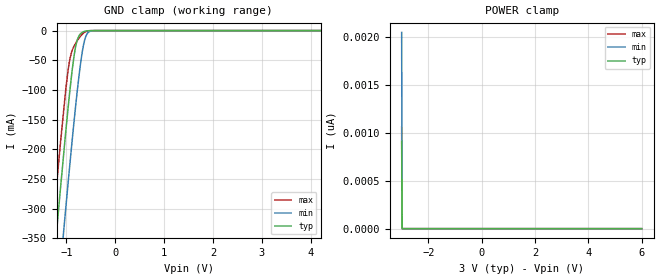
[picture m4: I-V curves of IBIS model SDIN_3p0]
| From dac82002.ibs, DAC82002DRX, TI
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|   Model
[Model]   SDIN_3p0
Model_type   Input
Vinl = 0.9
Vinh = 2.1
|   typ   min   max
C_comp   3.377pF   3.057pF   3.504pF
[Voltage Range]   3   2.7   3.3
[Temperature Range]   25   125   -40
[Power Clamp Reference]   3   2.7   3.3
[GND Clamp Reference]   0   0   0
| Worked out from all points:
|   GND clamp passes 1 mA (typ) near -0.61 V on its own axis
[GND Clamp]
|   Voltage   I(typ)   I(min)   I(max)
-3V       -2.092A    -2.219A    -2.017A
-1.353V   -483.7mA   -616.1mA   -404.6mA
-1.182V   -323.5mA   -455.6mA   -245.3mA
-1.119V   -265.8mA   -397.3mA   -188.9mA
-1.011V   -170.2mA   -299.1mA   -99.41mA
-930mV    -103.4mA   -227.6mA   -49.25mA
-840mV    -41.78mA   -151.7mA   -25.95mA
-777mV    -15.92mA   -102.4mA   -17.11mA
-651mV    -2.067mA   -25.52mA   -4.429mA
-570mV    -384.2uA   -4.886mA   -894.8uA
-426mV    -8.62uA    -122uA     -11.74uA
6V        0A         0A         0A
[POWER Clamp]
|   Voltage   I(typ)   I(min)   I(max)
-3V       912.4pA    2.049nA    1.062nA
-2.982V   0A         0A         0A
-2.973V   0A         0A         0A
6V        0A         0A         0A
